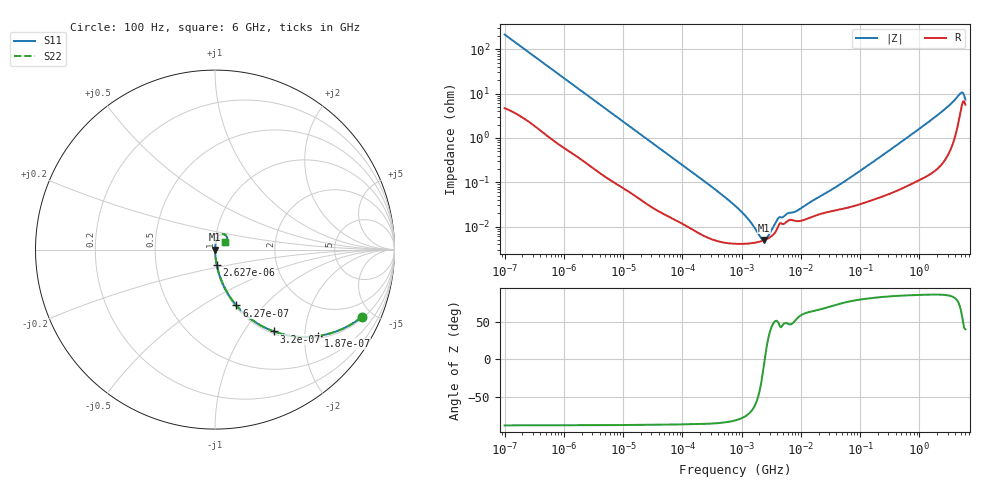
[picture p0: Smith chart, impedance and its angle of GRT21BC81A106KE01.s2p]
!Murata Part Number: GRT21BC81A106KE01
!These Parameters are Measured in Series Mode Connection
!Data Generated on Jun 19, 2026
!  o--ll--o
!Port1  Port2
!  o------o
!Operation Temp=25[degC], DC Bias Voltage=0[V]
!Freq. Start=100[Hz] Stop=6[GHz] 401[Steps]
# Hz S RI R 50
!Freq.(Hz) S11(Real) S11(Imag) S21(Real) S21(Imag) S12(Real) S12(Imag) S22(Real) S22(Imag)
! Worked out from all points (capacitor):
!   401 points, 100 Hz to 6 GHz, reference 50 ohm
!   read as one part in series: C = 7.33 uF near 109 Hz
!   lowest |Z| = 4.97 mohm at 2.373 MHz (marker M1)
!   series resonance near 2.464 MHz, so ESL is about 570 pH
!   S11 on the Smith chart (normalised r, x): 100 Hz: 1.09, -4.32; 187 Hz: 1.06, -2.33; 320 Hz: 1.04, -1.38; 627 Hz: 1.02, -0.71; 2.627 kHz: 1.00, -0.17; 6 GHz: 1.11, +0.09
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100  0.818 -0.3751  0.182 0.3751  0.182 0.3751  0.818 -0.3751
187  0.5748 -0.4814  0.4252 0.4814  0.4252 0.4814  0.5748 -0.4814
320  0.3267 -0.4557  0.6733 0.4557  0.6733 0.4557  0.3267 -0.4557
627  0.119 -0.311  0.881 0.311  0.881 0.311  0.119 -0.311
1026  0.0509 -0.207  0.9491 0.207  0.9491 0.207  0.0509 -0.207
2008  0.0158 -0.1113  0.9842 0.1113  0.9842 0.1113  0.0158 -0.1113
2627  0.00994 -0.0861  0.9901 0.0861  0.9901 0.0861  0.00994 -0.0861
40335  0.000255 -0.00597  0.9997 0.00597  0.9997 0.00597  0.000255 -0.00597
289253  5.48e-05 -0.000858  0.9999 0.000858  0.9999 0.000858  5.48e-05 -0.000858
774597  4.11e-05 -0.000295  1 0.000295  1 0.000295  4.11e-05 -0.000295
1585629  4.29e-05 -9.41e-05  1 9.41e-05  1 9.41e-05  4.29e-05 -9.41e-05
2372521  4.91e-05 -7.9e-06  1 7.9e-06  1 7.9e-06  4.91e-05 -7.9e-06
3245845  6.19e-05 6e-05  0.9999 -6e-05  0.9999 -6e-05  6.19e-05 6e-05
4440638  0.000119 0.000114  0.9999 -0.000114  0.9999 -0.000114  0.000119 0.000114
8311524  0.000133 0.000177  0.9999 -0.000177  0.9999 -0.000177  0.000133 0.000177
1.555665e7  0.000167 0.000342  0.9998 -0.000342  0.9998 -0.000342  0.000167 0.000342
5.211241e7  0.000254 0.000969  0.9997 -0.000969  0.9997 -0.000969  0.000254 0.000969
3.124326e8  0.000573 0.00521  0.9994 -0.00521  0.9994 -0.00521  0.000573 0.00521
2.048624e9  0.00312 0.0329  0.9969 -0.0329  0.9969 -0.0329  0.00312 0.0329
4.796499e9  0.0373 0.0861  0.9627 -0.0861  0.9627 -0.0861  0.0373 0.0861
5.245841e9  0.0596 0.081  0.9404 -0.081  0.9404 -0.081  0.0596 0.081
6e9  0.055 0.0421  0.945 -0.0421  0.945 -0.0421  0.055 0.0421
